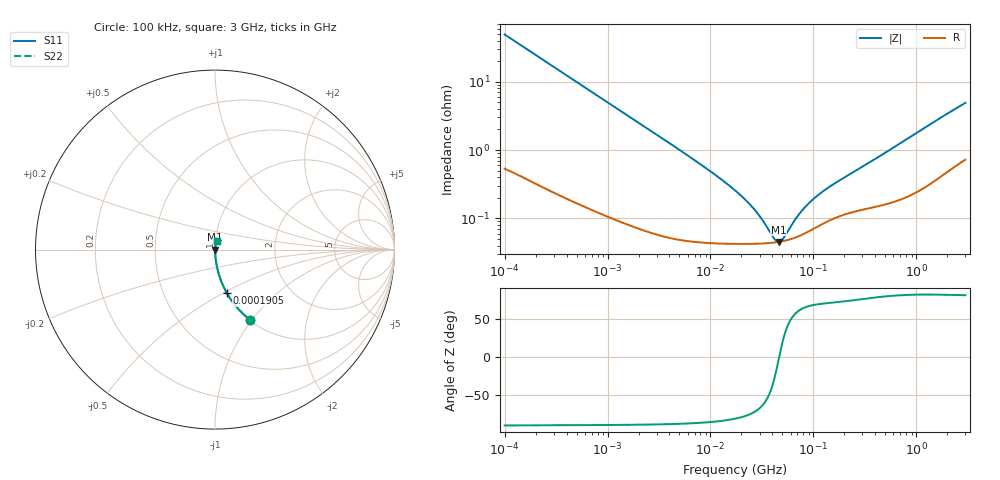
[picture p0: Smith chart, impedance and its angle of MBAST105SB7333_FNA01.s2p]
! MBAST105SB7333_FNA01  S-PARAMETER MODEL  ( Standard Model )
! Model Generated by TAIYO YUDEN Corporation (http://www.ty-top.com)
! Version 1.0
! TAIYO YUDEN Control No. 220601
! Copyright(c) 2017 TAIYO YUDEN CO.,LTD. All Rights Reserved.
! Product Description (link to TY-COMPAS)
! https://ds.yuden.co.jp/TYCOMPAS/or/detail?pn=MBAST105SB7333KFNA01&u=M
! Products Name : Multilayer Ceramic Capacitors
! Characteristics :
!  Capacitance : 0.033 [uF] , Rated Voltage : 25 [V] , TCC : X7R
!  Case Size : 1.0 x 0.5 / 0.039 x 0.02 [mm/inch] , Thickness : 0.5 / 0.02 [mm/inch]
!  (Conditions: Temperature = 25 [degC] , DC Bias Voltage = 0 [V])
! External Node Assignments :
!  1  o---| |---o  2
! GND o---------o GND
! Frequency Range : 100kHz  -  3GHz  [ 401 STEP ]
# MHZ S RI R 50
! Freq[MHz].  S11 Real  S11 Imag  S21 Real  S21 Imag  S12 Real  S12 Imag  S22 Real  S22 Imag
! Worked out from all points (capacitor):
!   401 points, 100 kHz to 3 GHz, reference 50 ohm
!   read as one part in series: C = 32.3 nF near 105.3 kHz
!   lowest |Z| = 45.2 mohm at 46.12 MHz (marker M1)
!   series resonance near 46.47 MHz, so ESL is about 360 pH
!   S11 on the Smith chart (normalised r, x): 100 kHz: 1.01, -0.98; 190.5 kHz: 1.01, -0.52; 3 GHz: 1.01, +0.10
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0.1  0.1974 -0.3927  0.8026 0.3927  0.8026 0.3927  0.1974 -0.3927
0.1398  0.1136 -0.3114  0.8864 0.3114  0.8864 0.3114  0.1136 -0.3114
0.190467  0.0658 -0.2416  0.9342 0.2416  0.9342 0.2416  0.0658 -0.2416
0.318916  0.0257 -0.1513  0.9743 0.1513  0.9743 0.1513  0.0257 -0.1513
0.562235  0.0093 -0.0877  0.9907 0.0877  0.9907 0.0877  0.0093 -0.0877
1.18716  0.00273 -0.0421  0.9973 0.0421  0.9973 0.0421  0.00273 -0.0421
3.161081  0.000819 -0.0159  0.9992 0.0159  0.9992 0.0159  0.000819 -0.0159
9.574722  0.000461 -0.00509  0.9995 0.00509  0.9995 0.00509  0.000461 -0.00509
17.7727  0.000428 -0.00245  0.9996 0.00245  0.9996 0.00245  0.000428 -0.00245
22.41241  0.000425 -0.00175  0.9996 0.00175  0.9996 0.00175  0.000425 -0.00175
26.84345  0.000426 -0.00127  0.9996 0.00127  0.9996 0.00127  0.000426 -0.00127
32.15051  0.000429 -0.00083  0.9996 0.00083  0.9996 0.00083  0.000429 -0.00083
41.60216  0.000442 -0.000245  0.9996 0.000245  0.9996 0.000245  0.000442 -0.000245
43.80277  0.000447 -0.00013  0.9996 0.00013  0.9996 0.00013  0.000447 -0.00013
46.11977  0.000452 -1.65e-05  0.9995 1.65e-05  0.9995 1.65e-05  0.000452 -1.65e-05
51.12795  0.000465 0.000212  0.9995 -0.000212  0.9995 -0.000212  0.000465 0.000212
71.47675  0.000545 0.000972  0.9995 -0.000972  0.9995 -0.000972  0.000545 0.000972
97.38194  0.000688 0.00172  0.9993 -0.00172  0.9993 -0.00172  0.000688 0.00172
150.9232  0.000972 0.00289  0.999 -0.00289  0.999 -0.00289  0.000972 0.00289
547.5153  0.00175 0.00979  0.9982 -0.00979  0.9982 -0.00979  0.00175 0.00979
1701.687  0.00482 0.0288  0.9952 -0.0288  0.9952 -0.0288  0.00482 0.0288
3000  0.00947 0.0477  0.9905 -0.0477  0.9905 -0.0477  0.00947 0.0477
